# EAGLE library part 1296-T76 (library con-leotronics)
1.27mm SINGLE ROW FEMALE SOCKET Source: http://www.leotronics.co.uk/Conexcon/Data%20Sheets/sec.%20A/1296ing.pdf
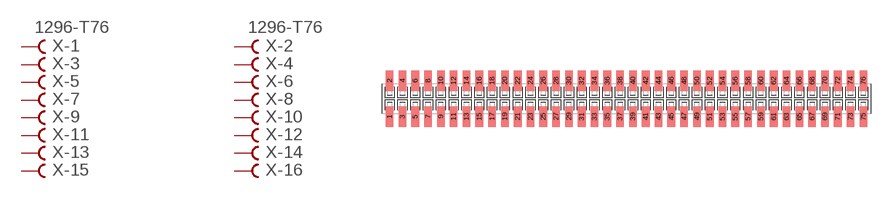
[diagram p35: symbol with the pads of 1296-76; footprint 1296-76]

Designator prefix X; gates -1=FVAL -2=FVAL -3=F -4=F -5=F -6=F -7=F -8=F -9=F -10=F -11=F -12=F -13=F -14=F -15=F -16=F -17=F -18=F -19=F -20=F -21=F -22=F -23=F -24=F -25=F -26=F -27=F -28=F -29=F -30=F -31=F -32=F -33=F -34=F -35=F -36=F -37=F -38=F -39=F -40=F -41=F -42=F -43=F -44=F -45=F -46=F -47=F -48=F -49=F -50=F -51=F -52=F -53=F -54=F -55=F -56=F -57=F -58=F -59=F -60=F -61=F -62=F -63=F -64=F -65=F -66=F -67=F -68=F -69=F -70=F -71=F -72=F -73=F -74=F -75=F -76=F

## 1296-T76 (OC_FARNELL: unknown; OC_NEWARK: unknown)  [1296-76]
1  -1:B  pas
2  -2:B  pas
3  -3:B  pas
4  -4:B  pas
5  -5:B  pas
6  -6:B  pas
7  -7:B  pas
8  -8:B  pas
9  -9:B  pas
10  -10:B  pas
11  -11:B  pas
12  -12:B  pas
13  -13:B  pas
14  -14:B  pas
15  -15:B  pas
16  -16:B  pas
17  -17:B  pas
18  -18:B  pas
19  -19:B  pas
20  -20:B  pas
21  -21:B  pas
22  -22:B  pas
23  -23:B  pas
24  -24:B  pas
25  -25:B  pas
26  -26:B  pas
27  -27:B  pas
28  -28:B  pas
29  -29:B  pas
30  -30:B  pas
31  -31:B  pas
32  -32:B  pas
33  -33:B  pas
34  -34:B  pas
35  -35:B  pas
36  -36:B  pas
37  -37:B  pas
38  -38:B  pas
39  -39:B  pas
40  -40:B  pas
41  -41:B  pas
42  -42:B  pas
43  -43:B  pas
44  -44:B  pas
45  -45:B  pas
46  -46:B  pas
47  -47:B  pas
48  -48:B  pas
49  -49:B  pas
50  -50:B  pas
51  -51:B  pas
52  -52:B  pas
53  -53:B  pas
54  -54:B  pas
55  -55:B  pas
56  -56:B  pas
57  -57:B  pas
58  -58:B  pas
59  -59:B  pas
60  -60:B  pas
61  -61:B  pas
62  -62:B  pas
63  -63:B  pas
64  -64:B  pas
65  -65:B  pas
66  -66:B  pas
67  -67:B  pas
68  -68:B  pas
69  -69:B  pas
70  -70:B  pas
71  -71:B  pas
72  -72:B  pas
73  -73:B  pas
74  -74:B  pas
75  -75:B  pas
76  -76:B  pas

## Footprint 1296-76 (pad centres in mm)
1.27mm SINGLE ROW FEMALE SOCKET Source: http://www.leotronics.co.uk/Conexcon/Data%20Sheets/sec.%20A/1296ing.pdf
smd 0.76 x 2.05: 1 -23.495,-1.78; 2 -23.495,1.78; 3 -22.225,-1.78; 4 -22.225,1.78; 5 -20.955,-1.78; 6 -20.955,1.78; 7 -19.685,-1.78; 8 -19.685,1.78; 9 -18.415,-1.78; 10 -18.415,1.78; 11 -17.145,-1.78; 12 -17.145,1.78; 13 -15.875,-1.78; 14 -15.875,1.78; 15 -14.605,-1.78; 16 -14.605,1.78; 17 -13.335,-1.78; 18 -13.335,1.78; 19 -12.065,-1.78; 20 -12.065,1.78; 21 -10.795,-1.78; 22 -10.795,1.78; 23 -9.525,-1.78; 24 -9.525,1.78; 25 -8.255,-1.78; 26 -8.255,1.78; 27 -6.985,-1.78; 28 -6.985,1.78; 29 -5.715,-1.78; 30 -5.715,1.78; 31 -4.445,-1.78; 32 -4.445,1.78; 33 -3.175,-1.78; 34 -3.175,1.78; 35 -1.905,-1.78; 36 -1.905,1.78; 37 -0.635,-1.78; 38 -0.635,1.78; 39 0.635,-1.78; 40 0.635,1.78; 41 1.905,-1.78; 42 1.905,1.78; 43 3.175,-1.78; 44 3.175,1.78; 45 4.445,-1.78; 46 4.445,1.78; 47 5.715,-1.78; 48 5.715,1.78; 49 6.985,-1.78; 50 6.985,1.78; 51 8.255,-1.78; 52 8.255,1.78; 53 9.525,-1.78; 54 9.525,1.78; 55 10.795,-1.78; 56 10.795,1.78; 57 12.065,-1.78; 58 12.065,1.78; 59 13.335,-1.78; 60 13.335,1.78; 61 14.605,-1.78; 62 14.605,1.78; 63 15.875,-1.78; 64 15.875,1.78; 65 17.145,-1.78; 66 17.145,1.78; 67 18.415,-1.78; 68 18.415,1.78; 69 19.685,-1.78; 70 19.685,1.78; 71 20.955,-1.78; 72 20.955,1.78; 73 22.225,-1.78; 74 22.225,1.78; 75 23.495,-1.78; 76 23.495,1.78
